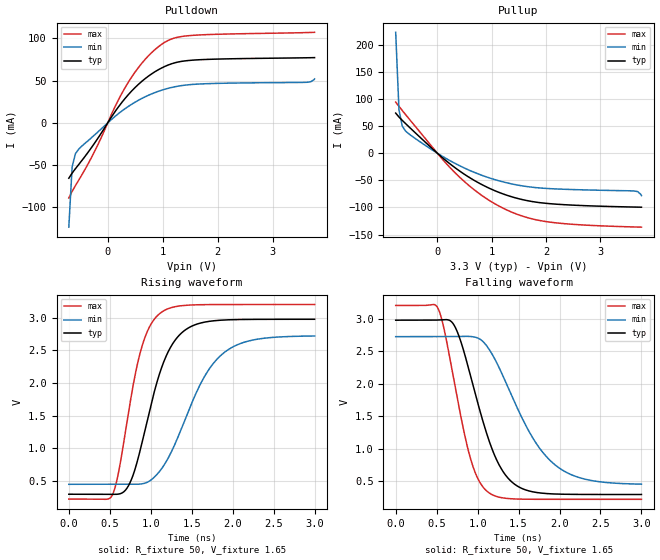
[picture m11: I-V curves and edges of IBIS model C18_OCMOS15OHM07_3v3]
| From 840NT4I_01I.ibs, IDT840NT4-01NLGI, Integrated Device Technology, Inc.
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| 4.00000e+00   -2.69859e-03   -1.00314e+00   -1.01762e-04
| 4.10000e+00   -1.68596e-02   -2.32449e+00   -1.11528e-03
| 4.20000e+00   -4.41704e-01   -3.64702e+00   -5.92810e-03
| 4.30000e+00   -2.03107e+00   -4.97033e+00   -1.62153e-02
| 4.40000e+00   -3.62163e+00   -6.29416e+00   -7.71540e-02
| 4.50000e+00   -5.21296e+00   -7.61836e+00   -1.59468e+00
| 4.60000e+00   -6.80478e+00   -8.94279e+00   -3.63022e+00
| 4.70000e+00   -8.39687e+00   -1.02674e+01   -5.66629e+00
| 4.80000e+00   -9.98911e+00   -1.15920e+01   -7.70259e+00
| 4.90000e+00   -1.15814e+01   -1.29167e+01   -9.73892e+00
| 5.00000e+00   -1.31736e+01   -1.42413e+01   -1.17752e+01
| 5.10000e+00   -1.47657e+01   -1.55659e+01   -1.38112e+01
| 5.20000e+00   -1.63577e+01   -1.68904e+01   -1.58470e+01
| 5.30000e+00   -1.79495e+01   -1.82147e+01   -1.78825e+01
| 5.40000e+00   -1.95411e+01   -1.95390e+01   -1.99177e+01
| 5.50000e+00   -2.11325e+01   -2.08630e+01   -2.19525e+01
| 5.60000e+00   -2.27236e+01   -2.21870e+01   -2.39869e+01
| 5.70000e+00   -2.43144e+01   -2.35107e+01   -2.60210e+01
| 5.80000e+00   -2.59051e+01   -2.48343e+01   -2.80547e+01
| 5.90000e+00   -2.74954e+01   -2.61577e+01   -3.00881e+01
| 6.00000e+00   -2.90855e+01   -2.74809e+01   -3.21210e+01
| 6.10000e+00   -3.06753e+01   -2.88039e+01   -3.41536e+01
| 6.20000e+00   -3.22648e+01   -3.01267e+01   -3.61858e+01
| 6.30000e+00   -3.38541e+01   -3.14494e+01   -3.82177e+01
| 6.40000e+00   -3.54431e+01   -3.27718e+01   -4.02492e+01
| 6.50000e+00   -3.70319e+01   -3.40941e+01   -4.22803e+01
| 6.60000e+00   -3.86204e+01   -3.54162e+01   -4.43110e+01
[Model] C18_OCMOS15OHM07_3v3
Model_type   Output
Polarity   Non-Inverting
|   typ   min   max
C_comp   2pF   1.5pF   2.5pF
Vmeas = 1.65V
Rref = 50
Cref = 0
Vref = 1.65V
|   typ   min   max
[Voltage range]   3.3V   3.135V   3.465V
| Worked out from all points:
|   slope of the pulldown table from 0 to 0.495 V, typ, clamps not added: 11.9 ohm
|   slope of the pullup table from 0 to 0.495 V, typ, clamps not added: 12.8 ohm
|   rising waveform, R_fixture 50, V_fixture 1.65: 20-80 % time 355ps typ, 508ps min, 270ps max; typ from 0.293 V to 2.98 V
|   falling waveform, R_fixture 50, V_fixture 1.65: 20-80 % time 386ps typ, 565ps min, 291ps max; typ from 2.98 V to 0.293 V
[Pulldown]
|Voltage   I (typ)   I (min)   I (max)
|Note, modeling breaks down at 250mA and above.  This is well beyond the functional   |
|operating range of the device.  Should this scenario occur, catastrophic failure and   |
|possible damage to the device and/or board is of higher concern than the I-V curve   |
|behavior.  The IBIS checker will flag currents in excess of 10A with warnings.  Lines   |
|with currents in excess of 0.35 A have been commented out.  The points still remain|
|available to the user if the user desires to use them.   |
|-2.94000e+00   -3.59168e+01   -2.87150e+01   -4.40479e+01
|-2.58000e+00   -2.96864e+01   -2.40476e+01   -3.60851e+01
|-2.22000e+00   -2.34518e+01   -1.93774e+01   -2.81172e+01
|-1.86000e+00   -1.72122e+01   -1.47039e+01   -2.01427e+01
|-1.50000e+00   -1.09669e+01   -1.00276e+01   -1.21595e+01
|-1.49000e+00   -1.07933e+01   -9.89764e+00   -1.19376e+01
|-1.42977e+00   -9.74797e+00   -9.11508e+00   -1.06011e+01
|-1.36954e+00   -8.70253e+00   -8.33248e+00   -9.26433e+00
|-1.30931e+00   -7.65701e+00   -7.54987e+00   -7.92740e+00
|-1.24908e+00   -6.61145e+00   -6.76726e+00   -6.59031e+00
|-1.18885e+00   -5.56588e+00   -5.98467e+00   -5.25310e+00
|-1.12862e+00   -4.52032e+00   -5.20211e+00   -3.91580e+00
|-1.06839e+00   -3.47482e+00   -4.41963e+00   -2.57847e+00
|-1.00816e+00   -2.42943e+00   -3.63723e+00   -1.24118e+00
|-9.47931e-01   -1.38423e+00   -2.85499e+00   -2.29472e-01
|-8.87701e-01   -3.76112e-01   -2.07295e+00   -1.24198e-01
|-8.27471e-01   -1.07547e-01   -1.29120e+00   -1.08395e-01
|-7.67241e-01   -7.45770e-02   -5.09851e-01   -9.79207e-02
-707mV    -65.46mA   -123.3mA   -88.8mA
-646.8mV  -59.42mA   -51.97mA   -81mA
-586.6mV  -54.19mA   -36.45mA   -74.17mA
-285.4mV  -28.3mA    -16.97mA   -39.73mA
136.2mV   13.58mA    7.833mA    19.64mA
377.1mV   33.56mA    19.57mA    48.34mA
678.3mV   52.24mA    30.8mA     74.98mA
979.4mV   64.93mA    38.64mA    92.89mA
1.22V     71.08mA    42.73mA    100.5mA
1.521V    74.09mA    45.39mA    103.4mA
3.63V     77.03mA    48.08mA    106.8mA
3.76V     77.21mA    52mA       107.1mA
| 4.32800e+00   2.24435e+00   5.40928e+00   1.18398e-01
| 4.89600e+00   1.17779e+01   1.25505e+01   9.83217e+00
| 5.46400e+00   2.13261e+01   1.97034e+01   2.20412e+01
| 6.03200e+00   3.08942e+01   2.68763e+01   3.42728e+01
| 6.60000e+00   4.04978e+01   3.40931e+01   4.65391e+01
[Pullup]
|Voltage   I (typ)   I (min)   I (max)
|Note, modeling breaks down at 250mA and above.  This is well beyond the functional   |
|operating range of the device.  Should this scenario occur, catastrophic failure and   |
|possible damage to the device and/or board is of higher concern than the I-V curve   |
|behavior.  The IBIS checker will flag currents in excess of 10A with warnings.  Lines   |
|with currents in excess of 0.35 A have been commented out.  The points still remain|
|available to the user if the user desires to use them.   |
|-2.94000e+00   3.45004e+01   2.75227e+01   4.23914e+01
|-2.58000e+00   2.84271e+01   2.29685e+01   3.46316e+01
|-2.22000e+00   2.23458e+01   1.84112e+01   2.68615e+01
|-1.86000e+00   1.62713e+01   1.38569e+01   1.91001e+01
|-1.50000e+00   1.02033e+01   9.30915e+00   1.13450e+01
|-1.49000e+00   1.00348e+01   9.18289e+00   1.11296e+01
|-1.42977e+00   9.02011e+00   8.42256e+00   9.83258e+00
|-1.36954e+00   8.00552e+00   7.66235e+00   8.53567e+00
|-1.30931e+00   6.99103e+00   6.90226e+00   7.23885e+00
|-1.24908e+00   5.97665e+00   6.14228e+00   5.94212e+00
|-1.18885e+00   4.96237e+00   5.38241e+00   4.64548e+00
|-1.12862e+00   3.94819e+00   4.62263e+00   3.34892e+00
|-1.06839e+00   2.93409e+00   3.86296e+00   2.05244e+00
|-1.00816e+00   1.92009e+00   3.10338e+00   7.56040e-01
|-9.47931e-01   9.06176e-01   2.34389e+00   1.55664e-01
|-8.87701e-01   1.92152e-01   1.58450e+00   1.12026e-01
|-8.27471e-01   9.02170e-02   8.25201e-01   1.02083e-01
-767.2mV  73.92mA    222.7mA    94.12mA
-707mV    66.71mA    80.24mA    86.37mA
-646.8mV  60.57mA    50.13mA    78.76mA
-526.3mV  48.91mA    35.69mA    63.96mA
-164.9mV  15.08mA    10.69mA    20.1mA
256.7mV   -21.49mA   -15.08mA   -28.91mA
618mV     -46.44mA   -32.66mA   -62.5mA
979.4mV   -65.61mA   -46.21mA   -88.43mA
1.401V    -81.23mA   -57.23mA   -109.9mA
2.184V    -93.88mA   -65.83mA   -128.3mA
3.63V     -99.24mA   -69.66mA   -135.9mA
3.76V     -99.51mA   -78.15mA   -136.3mA
| 4.32800e+00   -2.79639e+00   -6.05511e+00   -1.58367e-01
| 4.89600e+00   -1.26437e+01   -1.34270e+01   -1.06532e+01
| 5.46400e+00   -2.24924e+01   -2.07986e+01   -2.32486e+01
| 6.03200e+00   -3.23378e+01   -2.81663e+01   -3.58417e+01
| 6.60000e+00   -4.21848e+01   -3.55299e+01   -4.84458e+01
[Ramp]
|   typ   min   max
dV/dt_r   1.611/0.355n   1.365/0.508n   1.793/0.269n
dV/dt_f   1.615/0.386n   1.365/0.565n   1.799/0.292n
R_load =   50.0000
[Rising Waveform]
R_fixture = 50
V_fixture = 1.65   |Vcc_typ
V_fixture_min = 1.5675 |Vcc_min
V_fixture_max = 1.7325 |Vcc_max
C_fixture = 0.0p
| Time   typ   min   max
0s        293.1mV    445.5mV    218.6mV
531.5ps   291.8mV    445.6mV    281.2mV
603.6ps   294.8mV    445.7mV    606.1mV
714.7ps   395.3mV    445.4mV    1.438V
867.9ps   951.5mV    448.3mV    2.448V
1.114ns   2.167V     654mV      3.069V
1.39ns    2.783V     1.348V     3.187V
1.64ns    2.929V     2.062V     3.201V
1.868ns   2.964V     2.436V     3.203V
3ns       2.977V     2.72V      3.203V
[Falling Waveform]
R_fixture = 50
V_fixture = 1.65   |Vcc_typ
V_fixture_min = 1.5675 |Vcc_min
V_fixture_max = 1.7325 |Vcc_max
C_fixture = 0.0p
| Time   typ   min   max
0s        2.977V     2.724V     3.203V
519.5ps   2.98V      2.724V     3.152V
747.7ps   2.81V      2.725V     1.801V
936.9ps   2.007V     2.723V     748mV
1.126ns   1.172V     2.555V     331.1mV
1.42ns    482.8mV    1.802V     226.4mV
1.679ns   332.9mV    1.153V     219.4mV
1.913ns   302.3mV    784.2mV    218.7mV
2.309ns   293.9mV    529.6mV    218.6mV
3ns       293.1mV    452.1mV    218.6mV
